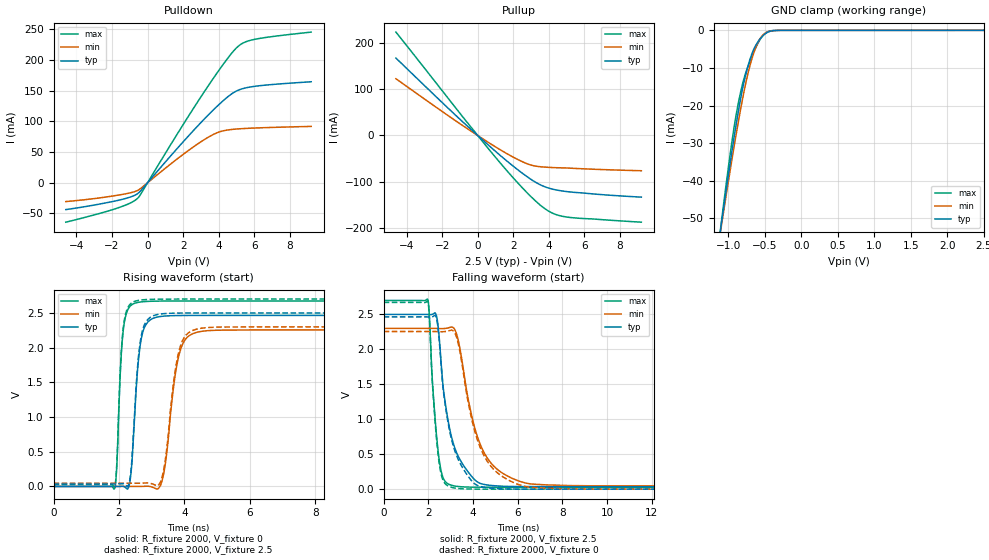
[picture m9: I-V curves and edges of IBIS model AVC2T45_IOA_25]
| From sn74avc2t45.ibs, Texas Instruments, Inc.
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[Model]   AVC2T45_IOA_25
Model_type  I/O
Vinl=0.7
Vinh=1.6
Enable   Active-Low
Vref =   0
Rref =   2000
Cref =   15p
Vmeas =   1.25
| variable   typ   min   max
C_comp   4.92pF   4.20pF   5.67pF
| C_pullup   4.12pF   3.15pF   5.54pF
| C_pulldown   4.24pF   3.76pF   4.71pF
| C_tri-state   4.92pF   4.20pF   5.67pF
[Temperature Range]   40   100   -40
| Ambient temperature   25   85   -40
[Voltage range]   2.5   2.3   2.7
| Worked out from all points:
|   slope of the pulldown table from 0 to 0.375 V, typ, clamps not added: 29.4 ohm
|   slope of the pullup table from 0 to 0.375 V, typ, clamps not added: 28.8 ohm
|   GND clamp passes 1 mA (typ) near -0.50 V on its own axis
|   rising waveform, R_fixture 2000, V_fixture 0: 20-80 % time 216ps typ, 341ps min, 152ps max; typ from 0 V to 2.46 V
|   falling waveform, R_fixture 2000, V_fixture 2.5: 20-80 % time 730ps typ, 1.04ns min, 339ps max; typ from 2.5 V to 0.036 V
|   rising waveform, R_fixture 2000, V_fixture 2.5: 20-80 % time 214ps typ, 337ps min, 151ps max; typ from 0.036 V to 2.5 V
|   falling waveform, R_fixture 2000, V_fixture 0: 20-80 % time 723ps typ, 1.04ns min, 331ps max; typ from 2.46 V to 0 V
[GND Clamp]
| AVC2T45_IOA_25
|   Voltage   I(typ)   I(min)   I(max)
-4.6V     -597.8mA   -546.6mA   -662.5mA
-1.105V   -52.8mA    -53.15mA   -52.37mA
-1.08V    -49.35mA   -50.03mA   -48.48mA
-930mV    -29.5mA    -31.88mA   -26.82mA
-880mV    -23.45mA   -26.17mA   -21.02mA
-825mV    -17.44mA   -20.22mA   -15.81mA
-750mV    -10.86mA   -13.03mA   -10.61mA
-665mV    -5.629mA   -6.786mA   -6.326mA
-580mV    -2.642mA   -2.683mA   -2.914mA
-500mV    -988.4uA   -823.5uA   -890.7uA
-280mV    -5.263uA   -7.282uA   -1.131uA
2.5V      1.201nA    548.8nA    148.6pA
[Pulldown]
| AVC2T45_IOA_25
|   Voltage   I(typ)   I(min)   I(max)
-4.6V     -43.76mA   -30.71mA   -64.27mA
-1.71V    -29.04mA   -20.44mA   -41.4mA
-985mV    -23.44mA   -16.53mA   -33.24mA
-545mV    -17.41mA   -12.35mA   -24.86mA
1.85V     61.76mA    42.85mA    87.78mA
3.295V    106.9mA    72.08mA    152.8mA
4.12V     130.1mA    83.49mA    187.5mA
4.755V    145.2mA    86.77mA    211.8mA
5.15V     151.2mA    87.75mA    223.4mA
5.55V     154.6mA    88.43mA    229.7mA
6.155V    157.4mA    89.2mA     234.2mA
9.2V      164.4mA    91.67mA    245.2mA
[Pullup]
| AVC2T45_IOA_25
|   Voltage   I(typ)   I(min)   I(max)
-4.6V     167.2mA    122.6mA    223.3mA
-1.155V   40.55mA    29.45mA    55.44mA
1.195V    -40.71mA   -29.18mA   -56.05mA
2.025V    -67.14mA   -47.36mA   -92.77mA
2.69V     -86.59mA   -59.63mA   -120.2mA
3.115V    -97.78mA   -65.03mA   -136.5mA
3.61V     -108mA     -67.79mA   -153.3mA
4.245V    -116.2mA   -69.29mA   -168.4mA
4.95V     -120.8mA   -70.1mA    -175.7mA
9.2V      -133.1mA   -76.13mA   -187.2mA
[Ramp]
| AVC2T45_IOA_25
| variable   typ   min   max
dV/dt_r   1.50/2.23E-10   1.38/3.53E-10   1.63/1.54E-10
dV/dt_f   1.49/7.29E-10   1.36/1.04E-09   1.62/3.41E-10
R_load = 2000
[Rising Waveform]
| AVC2T45_IOA_25
R_fixture =   2000
C_fixture =   0
L_fixture =   0
V_fixture =   0
V_fixture_min = 0
V_fixture_max = 0
|   Time   V(typ)   V(min)   V(max)
0s        27.74nV    106.5nV    1.06nV
1.87ns    22.36uV    -2.483uV   -26.64mV
2.14ns    969.3uV    -31.91uV   2.287V
2.355ns   141.5mV    38.27uV    2.604V
2.6ns     1.844V     -228.4uV   2.654V
2.785ns   2.299V     2.389mV    2.664V
3.27ns    2.449V     15.74mV    2.671V
3.845ns   2.463V     1.913V     2.672V
4.535ns   2.465V     2.236V     2.672V
34.99ns   2.465V     2.256V     2.672V
[Falling Waveform]
| AVC2T45_IOA_25
R_fixture =   2000
C_fixture =   0
L_fixture =   0
V_fixture =   2.5
V_fixture_min = 2.3
V_fixture_max = 2.7
|   Time   V(typ)   V(min)   V(max)
0s        2.5V       2.3V       2.7V
1.985ns   2.499V     2.3V       2.706V
2.21ns    2.506V     2.3V       1.403V
2.475ns   2.207V     2.298V     446.4mV
2.7ns     1.361V     2.298V     136.1mV
3.1ns     672.5mV    2.314V     50.63mV
3.98ns    166.8mV    994.8mV    29.02mV
4.41ns    73.9mV     576.6mV    28.03mV
6.345ns   36.64mV    87.92mV    27.63mV
34.99ns   36.05mV    46.86mV    27.62mV
[Rising Waveform]
| AVC2T45_IOA_25
R_fixture =   2000
C_fixture =   0
L_fixture =   0
V_fixture =   2.5
V_fixture_min = 2.3
V_fixture_max = 2.7
|   Time   V(typ)   V(min)   V(max)
0s        36.05mV    46.86mV    27.62mV
1.87ns    36.08mV    46.85mV    986.6uV
2.14ns    37.01mV    46.82mV    2.318V
2.355ns   179.1mV    46.89mV    2.632V
2.61ns    1.933V     46.65mV    2.682V
2.81ns    2.36V      49.83mV    2.692V
3.27ns    2.485V     64mV       2.699V
3.835ns   2.498V     1.954V     2.7V
4.51ns    2.5V       2.28V      2.7V
34.99ns   2.5V       2.3V       2.7V
[Falling Waveform]
| AVC2T45_IOA_25
R_fixture =   2000
C_fixture =   0
L_fixture =   0
V_fixture =   0
V_fixture_min = 0
V_fixture_max = 0
|   Time   V(typ)   V(min)   V(max)
0s        2.465V     2.256V     2.672V
1.985ns   2.464V     2.256V     2.678V
2.215ns   2.471V     2.256V     1.352V
2.47ns    2.189V     2.254V     408mV
2.695ns   1.343V     2.254V     104mV
3.08ns    658.5mV    2.273V     22.98mV
3.32ns    437.6mV    2.107V     10.47mV
4.4ns     32.43mV    537.1mV    386.7uV
6.3ns     517uV      40.76mV    13.72uV
34.99ns   386.2nV    342nV      223.9nV
